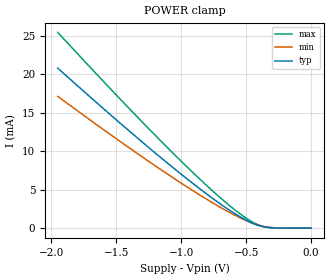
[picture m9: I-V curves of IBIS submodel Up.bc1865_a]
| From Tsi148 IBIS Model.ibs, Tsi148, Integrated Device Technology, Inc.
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[Submodel]  Up.bc1865_a
Submodel_type   Dynamic_clamp
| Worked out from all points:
|   POWER clamp passes 1 mA (typ) near -0.50 V on its own axis
[POWER Clamp]   | Note: Vtable = Vcc - Vout
| Voltage   I(typ)   I(min)   I(max)
-1.95V    20.79mA    17.12mA    25.44mA
-1.48V    13.79mA    11.39mA    16.96mA
-1.1V     8.378mA    6.963mA    10.37mA
-800mV    4.393mA    3.716mA    5.484mA
-580mV    1.817mA    1.621mA    2.289mA
-460mV    707uA      708uA      879uA
-360mV    157uA      212uA      170uA
-260mV    14uA       30uA       11uA
0V        0A         0A         0A
